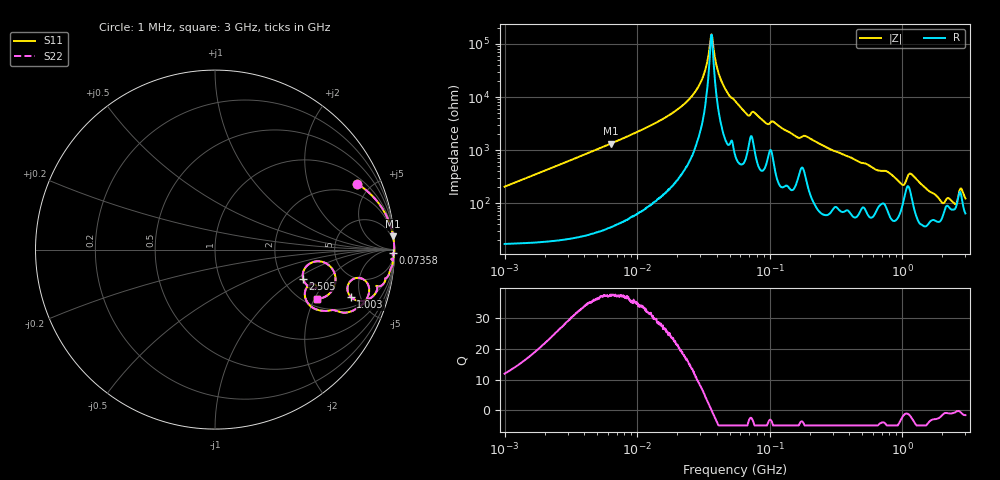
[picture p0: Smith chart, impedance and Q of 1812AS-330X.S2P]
!s-Parameter Generated by FASTRON Sdn. Bhd.
!FASTRON P/N : 1812AS-330X
!Keysight Technologies,E4991B,MY54100416,A.01.15
!Date created: Mon Oct 16 10:04:55 2023
!Version  : Rev00 Mon Oct 16 10:04:55 2023
!Data & Calibration Information:
!Freq	S11	S21	S12	S22
!PortZ  Port1:50+j0  Port2:50+j0
!When reading, reference impedance value at option line is always used.
! Remarks : This data is being provided solely for informational purposes.
# Hz S dB R 50
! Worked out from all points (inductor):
!   1601 points, 1 MHz to 3 GHz, reference 50 ohm
!   read as one part in series: L = 32.5 uH near 1.041 MHz
!   highest Q = 37.7 at 6.337 MHz (marker M1), where L = 33.4 uH
!   self-resonance near 36.34 MHz
!   S11 on the Smith chart (normalised r, x): 1 MHz: 1.34, +4.09; 73.58 MHz: open; 1.003 GHz: 2.78, -4.09; 2.505 GHz: 2.57, -1.13; 3 GHz: 2.29, -2.10
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1000000  -1.20 25.0  -7.45 -60.2  -7.45 -60.2  -1.20 25.0
3804036  -0.10 7.2  -17.99 -81.0  -17.99 -81.0  -0.10 7.2
6337400  -0.04 4.3  -22.51 -84.2  -22.51 -84.2  -0.04 4.3
1.447069e7  -0.01 1.7  -30.81 -86.4  -30.81 -86.4  -0.01 1.7
2.148682e7  -0.01 0.9  -36.39 -86.2  -36.39 -86.2  -0.01 0.9
2.773354e7  -0.01 0.4  -42.34 -84.3  -42.34 -84.3  -0.01 0.4
3.206477e7  -0.01 0.2  -48.89 -79.3  -48.89 -79.3  -0.01 0.2
3.633776e7  -0.01 0.0  -63.57 -5.6  -63.57 -5.6  -0.01 0.0
4.286213e7  -0.01 -0.3  -46.49 81.1  -46.49 81.1  -0.01 -0.3
5.477226e7  -0.01 -0.7  -38.56 83.8  -38.56 83.8  -0.01 -0.7
6.758263e7  -0.04 -1.2  -33.42 78.3  -33.42 78.3  -0.04 -1.2
7.358334e7  -0.06 -1.0  -34.39 69.3  -34.39 69.3  -0.06 -1.0
1.606197e8  -0.08 -3.2  -25.01 78.6  -25.01 78.6  -0.08 -3.2
2.083556e8  -0.06 -3.6  -24.03 82.0  -24.03 82.0  -0.06 -3.6
7.925923e8  -0.63 -14.0  -12.21 66.6  -12.21 66.6  -0.63 -14.0
1.002744e9  -1.93 -19.2  -8.90 47.3  -8.90 47.3  -1.93 -19.2
1.147801e9  -1.27 -12.2  -12.43 49.6  -12.43 49.6  -1.27 -12.2
1.557514e9  -1.96 -26.1  -6.91 51.1  -6.91 51.1  -1.96 -26.1
2.01032e9  -4.81 -28.6  -4.94 29.1  -4.94 29.1  -4.81 -28.6
2.505452e9  -5.73 -18.3  -5.44 17.6  -5.44 17.6  -5.73 -18.3
2.75535e9  -3.36 -11.3  -8.89 21.8  -8.89 21.8  -3.36 -11.3
3e9  -4.00 -25.9  -5.80 32.6  -5.80 32.6  -4.00 -25.9
